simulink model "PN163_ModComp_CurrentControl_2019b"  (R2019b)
settings: Solver=VariableStepAuto  StartTime=0.0  StopTime=0.04  RelTol=1e-3
PostLoadFcn:
  | run('PN163_param.m');
model workspace (MAT data in the model file):
  CTRLPERIOD = [5e-05 2.5001e-05]
  global_cycle_delay = 1e-05
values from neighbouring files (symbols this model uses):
  C = 260e-6    (= 0.00026)    [PN163_param.m]
  fs = 20e3    (= 20000)    [PN163_param.m]
  ki = 1/Ti1    (= 165)    [PN163_param.m]
  kp = Tn1/Ti1    (= 18.75)    [PN163_param.m]
  Lb = 2.5e-3    (= 0.0025)    [PN163_param.m]
  Rb = 22e-3    (= 0.022)    [PN163_param.m]
  Rload = 5    [PN163_param.m]
  SAMPLEPERIOD = [Ts Ts*phase]    [PN163_param.m]
  Ts = 1/fs    (= 5e-05)    [PN163_param.m]
  Vb = 100    [PN163_param.m]
undefined symbols (not defined in the file or in its folder): A, AXI4, bit, code, DiscIntNeverNeededParam, HLS, N, Stream, Top, width, xc7z030fbg676
libraries: ModelComposer x42, powerlib x24, powerlib_meascontrol x2

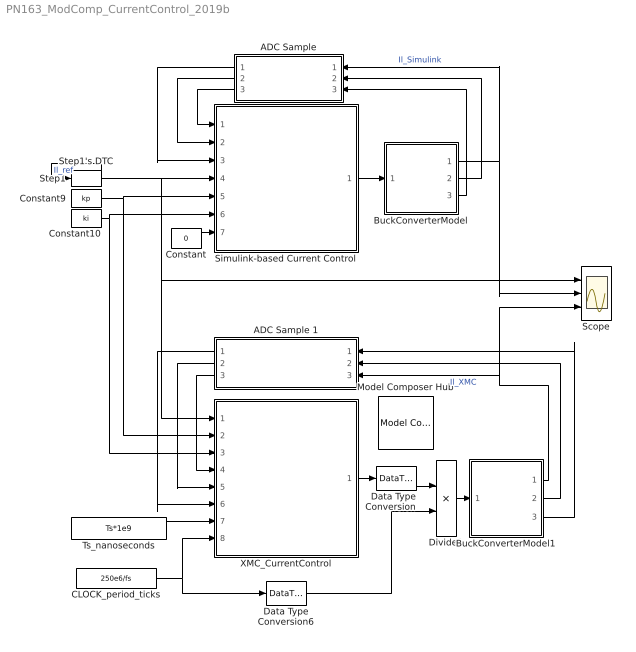
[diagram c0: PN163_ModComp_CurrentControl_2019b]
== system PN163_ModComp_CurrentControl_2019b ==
  ADC Sample : Subsystem
  ADC Sample 1 : Subsystem
  BuckConverterModel : Subsystem
  BuckConverterModel1 : Subsystem
  CLOCK_period_ticks : Constant  Value=250e6/fs  OutDataTypeStr=uint16  SampleTime=SAMPLEPERIOD
  Constant : Constant  Value=0  OutDataTypeStr=Inherit: Inherit via back propagation
  Constant10 : Constant  Value=ki  OutDataTypeStr=single  SampleTime=SAMPLEPERIOD
  Constant9 : Constant  Value=kp  OutDataTypeStr=single  SampleTime=SAMPLEPERIOD
  Data Type Conversion : DataTypeConversion  OutDataTypeStr=double
  Data Type Conversion6 : DataTypeConversion  OutDataTypeStr=double
  Divide1 : Product  Inputs=*/
  Model Composer Hub : ModelComposer/Model Composer Hub  CodeGeneration=off  SubsystemName=XMC_CurrentControl  TargetDirectory=C:/KB/PN163/Generated/Code  ExportType=HLS C++ code  IpVendor=xilinx.com  IpLibrary=hls  IpVersion=1.0  IpHWLanguage=Verilog  AieCompilerOptions={}  CreateTestbench=off  TestbenchStackSize=10  RunAieSim=off  AieSimTimeout=50000  LaunchVitisAnalyzer=off  RunX86Sim=off  X86SimTimeout=10  ProjDevice=xc7z030fbg676-3  ProjDevicePart=xc7z030fbg676-3  SamplePeriod=-1  ClockFrequency=250  DataPathParallelism=1
  Scope : Scope  NumInputPorts=3
  Simulink-based Current Control : Subsystem
  Step1 : Step  Time=0.02  Before=3  After=5  SampleTime=SAMPLEPERIOD
  Step1's DTC : DataTypeConversion
  Ts_nanoseconds : Constant  Value=Ts*1e9  OutDataTypeStr=uint32  SampleTime=SAMPLEPERIOD
  XMC_CurrentControl : Subsystem
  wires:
  BuckConverterModel/1(I) -> ADC Sample/1(Il_in), Scope/2  "Il_Simulink"
  Ts_nanoseconds/1 -> XMC_CurrentControl/7(Ts)
  Constant9/1 -> XMC_CurrentControl/2(Kp), Simulink-based Current Control/5(Kp)
  Constant10/1 -> Simulink-based Current Control/6(Ki), XMC_CurrentControl/3(Ki)
  XMC_CurrentControl/1(duty_cycle_ticks) -> Data Type Conversion/1
  Divide1/1 -> BuckConverterModel1/1(duty_cycle)
  ADC Sample 1/3(I_raw_int16) -> XMC_CurrentControl/4(Il_raw)
  ADC Sample 1/2(Vin_raw_int16) -> XMC_CurrentControl/5(Vin_raw)
  ADC Sample 1/1(Vout_raw_int16) -> XMC_CurrentControl/6(Vout_raw)
  BuckConverterModel1/3(Vout) -> ADC Sample 1/1(Vout_single)
  BuckConverterModel1/2(Vin) -> ADC Sample 1/2(Vin_single)
  BuckConverterModel1/1(I) -> Scope/3, ADC Sample 1/3(I_single)  "Il_XMC"
  Data Type Conversion/1 -> Divide1/1
  CLOCK_period_ticks/1 -> Data Type Conversion6/1, XMC_CurrentControl/8(CLOCK_period)
  Data Type Conversion6/1 -> Divide1/2
  Constant/1 -> Simulink-based Current Control/7(reset)
  Simulink-based Current Control/1(duty_cycle) -> BuckConverterModel/1(duty_cycle)
  BuckConverterModel/2(Vin) -> ADC Sample/2(Vin_in)
  BuckConverterModel/3(Vout) -> ADC Sample/3(vout_in)
  ADC Sample/3(Vout) -> Simulink-based Current Control/1(Vout)
  ADC Sample/2(Vin) -> Simulink-based Current Control/2(Vin)
  ADC Sample/1(Il) -> Simulink-based Current Control/3(Il)
  Step1/1 -> Step1's DTC/1  "Il_ref"
  Step1's DTC/1 -> XMC_CurrentControl/1(Il_ref), Scope/1, Simulink-based Current Control/4(I_ref)

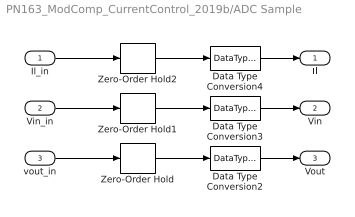
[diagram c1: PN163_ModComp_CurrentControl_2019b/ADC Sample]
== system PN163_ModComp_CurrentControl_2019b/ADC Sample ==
  Il_in : Inport
  Vin_in : Inport  Port=2
  vout_in : Inport  Port=3
  Data Type Conversion2 : DataTypeConversion  OutDataTypeStr=single
  Data Type Conversion3 : DataTypeConversion  OutDataTypeStr=single
  Data Type Conversion4 : DataTypeConversion  OutDataTypeStr=single
  Zero-Order Hold : ZeroOrderHold  SampleTime=SAMPLEPERIOD
  Zero-Order Hold1 : ZeroOrderHold  SampleTime=SAMPLEPERIOD
  Zero-Order Hold2 : ZeroOrderHold  SampleTime=SAMPLEPERIOD
  Il : Outport
  Vin : Outport  Port=2
  Vout : Outport  Port=3
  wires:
  Il_in/1 -> Zero-Order Hold2/1
  Data Type Conversion2/1 -> Vout/1
  Zero-Order Hold2/1 -> Data Type Conversion4/1
  Zero-Order Hold/1 -> Data Type Conversion2/1
  Vin_in/1 -> Zero-Order Hold1/1
  Zero-Order Hold1/1 -> Data Type Conversion3/1
  vout_in/1 -> Zero-Order Hold/1
  Data Type Conversion4/1 -> Il/1
  Data Type Conversion3/1 -> Vin/1

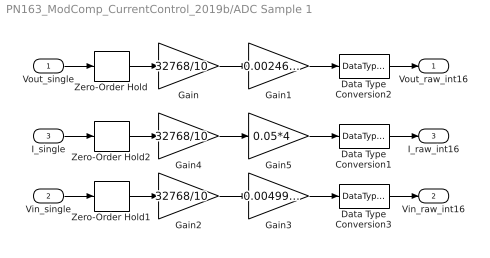
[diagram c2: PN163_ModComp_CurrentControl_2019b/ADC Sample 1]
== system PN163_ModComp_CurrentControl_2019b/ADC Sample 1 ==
  Vout_single : Inport
  Vin_single : Inport  Port=2
  I_single : Inport  Port=3
  Data Type Conversion1 : DataTypeConversion  OutDataTypeStr=int16
  Data Type Conversion2 : DataTypeConversion  OutDataTypeStr=int16
  Data Type Conversion3 : DataTypeConversion  OutDataTypeStr=int16
  Gain : Gain  Gain=32768/10
  Gain1 : Gain  Gain=0.00246*4
  Gain2 : Gain  Gain=32768/10
  Gain3 : Gain  Gain=0.00499*4
  Gain4 : Gain  Gain=32768/10
  Gain5 : Gain  Gain=0.05*4
  Zero-Order Hold : ZeroOrderHold  SampleTime=SAMPLEPERIOD
  Zero-Order Hold1 : ZeroOrderHold  SampleTime=SAMPLEPERIOD
  Zero-Order Hold2 : ZeroOrderHold  SampleTime=SAMPLEPERIOD
  Vout_raw_int16 : Outport
  Vin_raw_int16 : Outport  Port=2
  I_raw_int16 : Outport  Port=3
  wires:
  Vout_single/1 -> Zero-Order Hold/1
  Zero-Order Hold/1 -> Gain/1
  Gain/1 -> Gain1/1
  Data Type Conversion2/1 -> Vout_raw_int16/1
  Gain1/1 -> Data Type Conversion2/1
  Data Type Conversion3/1 -> Vin_raw_int16/1
  Gain3/1 -> Data Type Conversion3/1
  Zero-Order Hold1/1 -> Gain2/1
  Vin_single/1 -> Zero-Order Hold1/1
  Gain2/1 -> Gain3/1
  Gain4/1 -> Gain5/1
  I_single/1 -> Zero-Order Hold2/1
  Zero-Order Hold2/1 -> Gain4/1
  Gain5/1 -> Data Type Conversion1/1
  Data Type Conversion1/1 -> I_raw_int16/1

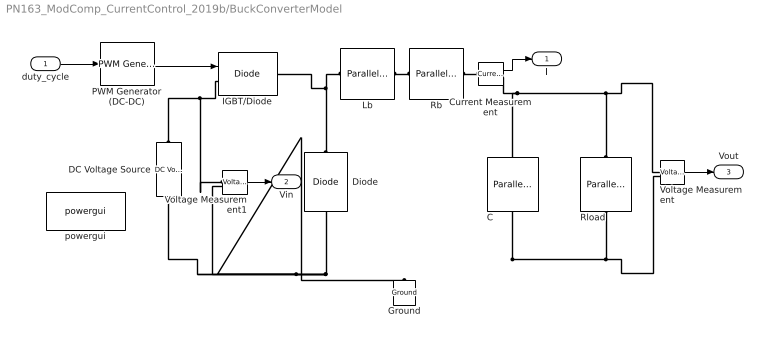
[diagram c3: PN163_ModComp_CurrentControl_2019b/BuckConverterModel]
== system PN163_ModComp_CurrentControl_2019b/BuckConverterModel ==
  duty_cycle : Inport
  C : powerlib/Elements/Parallel RLC Branch  LConnTagsString=a  RConnTagsString=__new0  BranchType=C  Resistance=5  Inductance=1e-3  SetiL0=off  InitialCurrent=0  Capacitance=C  Setx0=off  InitialVoltage=0  Measurements=None
  Current Measurement : powerlib/Measurements/Current Measurement  PhasorSimulation=off  OutputType=Complex  PSBequivalent=0
  DC Voltage Source : powerlib/Electrical Sources/DC Voltage Source  Amplitude=Vb  Measurements=Voltage
  Diode : powerlib/Power Electronics/Diode  Ron=0.001  Lon=0  Vf=0.8  IC=0  UseSnubber=0  Rs=500  Cs=250e-9  Measurements=off
  Ground : powerlib/Elements/Ground  LConnTagsString=a
  IGBT/Diode : powerlib/Power Electronics/IGBT//Diode  Ron=1e-3  Rs=1e5  Cs=inf  Measurements=off
  Lb : powerlib/Elements/Parallel RLC Branch  LConnTagsString=a  RConnTagsString=__new0  BranchType=L  Resistance=5  Inductance=Lb  SetiL0=off  InitialCurrent=0  Capacitance=1e-6  Setx0=off  InitialVoltage=0  Measurements=None
  PWM Generator (DC-DC) : powerlib_meascontrol/Pulse & Signal Generators/PWM Generator (DC-DC)  Fsw=fs  Ts=0
  Rb : powerlib/Elements/Parallel RLC Branch  LConnTagsString=a  RConnTagsString=__new0  BranchType=R  Resistance=Rb  Inductance=1e-3  SetiL0=off  InitialCurrent=0  Capacitance=1e-6  Setx0=off  InitialVoltage=0  Measurements=None
  Rload : powerlib/Elements/Parallel RLC Branch  LConnTagsString=a  RConnTagsString=__new0  BranchType=R  Resistance=Rload  Inductance=1e-3  SetiL0=off  InitialCurrent=0  Capacitance=1e-6  Setx0=off  InitialVoltage=0  Measurements=None
  Voltage Measurement : powerlib/Measurements/Voltage Measurement  PhasorSimulation=off  OutputType=Complex  PSBequivalent=0
  Voltage Measurement1 : powerlib/Measurements/Voltage Measurement  PhasorSimulation=off  OutputType=Complex  PSBequivalent=0
  powergui : powerlib/powergui  Priority=1  SimulationMode=Continuous  SampleTime=50e-6  frequency=60  Iterations=50  frequencyindice=0  Pbase=100e6  ErrMax=1e-4  UnitsV=kV  UnitsW=MW  buscounter=0  FunctionMessages=off  echomessages=off  EnableUseOfTLC=off  CurrentSourceSwitches=off  DisableSnubberDevices=off  DisableRonSwitches=off  DisableVfSwitches=off  DisplayEquations=off  AutomaticDiscreteSolvers=off  SolverType=Tustin/Backward Euler (TBE)  Interpol=off  ExternalGateDelay=off  methode=off  Ts=100  x0status=blocks  SPID=on  SwTol=0  HookPort=off  NonlinearTolerance=1e-4  nMaxIteration=100  ContinueOnMaxIteration=off  RestoreLinks=warning  ResistiveCurrentMeasurement=off  Frange=[0:2:500]  Ylog=off  Xlog=on  ShowGrid=off  save=off  variable=ZData  structure=0  ZoomFFT=off  StartTime=0.0  cycles=1  DisplayStyle=1  fundamental=60  FreqAxis=off  MaxFrequency=1000  frequencyindicesteady=1  RmsSteady=1  display=off
  I : Outport
  Vin : Outport  Port=2
  Vout : Outport  Port=3
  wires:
  duty_cycle/1 -> PWM Generator (DC-DC)/1
  Current Measurement/1 -> I/1
  Voltage Measurement1/1 -> Vin/1
  Voltage Measurement/1 -> Vout/1
  PWM Generator (DC-DC)/1 -> IGBT/Diode/1
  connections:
  Rload/RConn1 -- C/RConn1 -- DC Voltage Source/LConn1 -- Voltage Measurement1/LConn2 -- Diode/LConn1 -- Ground/LConn1 -- Voltage Measurement/LConn2
  DC Voltage Source/RConn1 -- IGBT/Diode/LConn1 -- Voltage Measurement1/LConn1
  Rload/LConn1 -- Current Measurement/RConn1 -- C/LConn1 -- Voltage Measurement/LConn1
  Lb/RConn1 -- Rb/LConn1
  Diode/RConn1 -- Lb/LConn1 -- IGBT/Diode/RConn1
  Rb/RConn1 -- Current Measurement/LConn1

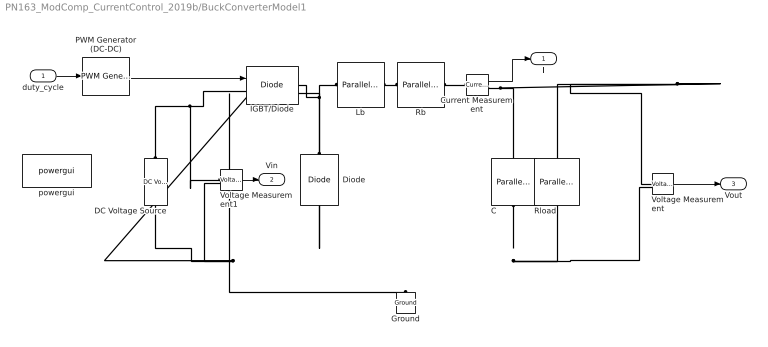
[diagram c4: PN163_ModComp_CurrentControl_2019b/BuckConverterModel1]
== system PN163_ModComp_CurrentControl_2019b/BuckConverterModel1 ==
  duty_cycle : Inport
  C : powerlib/Elements/Parallel RLC Branch  LConnTagsString=a  RConnTagsString=__new0  BranchType=C  Resistance=5  Inductance=1e-3  SetiL0=off  InitialCurrent=0  Capacitance=C  Setx0=off  InitialVoltage=0  Measurements=None
  Current Measurement : powerlib/Measurements/Current Measurement  PhasorSimulation=off  OutputType=Complex  PSBequivalent=0
  DC Voltage Source : powerlib/Electrical Sources/DC Voltage Source  Amplitude=Vb  Measurements=Voltage
  Diode : powerlib/Power Electronics/Diode  Ron=0.001  Lon=0  Vf=0.8  IC=0  UseSnubber=0  Rs=500  Cs=250e-9  Measurements=off
  Ground : powerlib/Elements/Ground  LConnTagsString=a
  IGBT/Diode : powerlib/Power Electronics/IGBT//Diode  Ron=1e-3  Rs=1e5  Cs=inf  Measurements=off
  Lb : powerlib/Elements/Parallel RLC Branch  LConnTagsString=a  RConnTagsString=__new0  BranchType=L  Resistance=5  Inductance=Lb  SetiL0=off  InitialCurrent=0  Capacitance=1e-6  Setx0=off  InitialVoltage=0  Measurements=None
  PWM Generator (DC-DC) : powerlib_meascontrol/Pulse & Signal Generators/PWM Generator (DC-DC)  Fsw=fs  Ts=0
  Rb : powerlib/Elements/Parallel RLC Branch  LConnTagsString=a  RConnTagsString=__new0  BranchType=R  Resistance=Rb  Inductance=1e-3  SetiL0=off  InitialCurrent=0  Capacitance=1e-6  Setx0=off  InitialVoltage=0  Measurements=None
  Rload : powerlib/Elements/Parallel RLC Branch  LConnTagsString=a  RConnTagsString=__new0  BranchType=R  Resistance=Rload  Inductance=1e-3  SetiL0=off  InitialCurrent=0  Capacitance=1e-6  Setx0=off  InitialVoltage=0  Measurements=None
  Voltage Measurement : powerlib/Measurements/Voltage Measurement  PhasorSimulation=off  OutputType=Complex  PSBequivalent=0
  Voltage Measurement1 : powerlib/Measurements/Voltage Measurement  PhasorSimulation=off  OutputType=Complex  PSBequivalent=0
  powergui : powerlib/powergui  Priority=1  SimulationMode=Continuous  SampleTime=50e-6  frequency=60  Iterations=50  frequencyindice=0  Pbase=100e6  ErrMax=1e-4  UnitsV=kV  UnitsW=MW  buscounter=0  FunctionMessages=off  echomessages=off  EnableUseOfTLC=off  CurrentSourceSwitches=off  DisableSnubberDevices=off  DisableRonSwitches=off  DisableVfSwitches=off  DisplayEquations=off  AutomaticDiscreteSolvers=off  SolverType=Tustin/Backward Euler (TBE)  Interpol=off  ExternalGateDelay=off  methode=off  Ts=100  x0status=blocks  SPID=on  SwTol=0  HookPort=off  NonlinearTolerance=1e-4  nMaxIteration=100  ContinueOnMaxIteration=off  RestoreLinks=warning  ResistiveCurrentMeasurement=off  Frange=[0:2:500]  Ylog=off  Xlog=on  ShowGrid=off  save=off  variable=ZData  structure=0  ZoomFFT=off  StartTime=0.0  cycles=1  DisplayStyle=1  fundamental=60  FreqAxis=off  MaxFrequency=1000  frequencyindicesteady=1  RmsSteady=1  display=off
  I : Outport
  Vin : Outport  Port=2
  Vout : Outport  Port=3
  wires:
  duty_cycle/1 -> PWM Generator (DC-DC)/1
  Current Measurement/1 -> I/1
  Voltage Measurement1/1 -> Vin/1
  Voltage Measurement/1 -> Vout/1
  PWM Generator (DC-DC)/1 -> IGBT/Diode/1
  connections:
  C/RConn1 -- Rload/RConn1 -- Voltage Measurement/LConn2 -- Voltage Measurement1/LConn2 -- DC Voltage Source/LConn1 -- Diode/LConn1 -- Ground/LConn1
  DC Voltage Source/RConn1 -- Voltage Measurement1/LConn1 -- IGBT/Diode/LConn1
  Current Measurement/RConn1 -- C/LConn1 -- Voltage Measurement/LConn1 -- Rload/LConn1
  Lb/RConn1 -- Rb/LConn1
  Diode/RConn1 -- IGBT/Diode/RConn1 -- Lb/LConn1
  Rb/RConn1 -- Current Measurement/LConn1

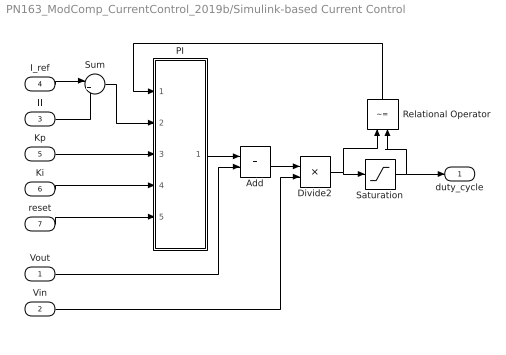
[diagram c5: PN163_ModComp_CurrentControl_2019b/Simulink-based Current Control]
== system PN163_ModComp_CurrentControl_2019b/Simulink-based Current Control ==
  Vout : Inport
  Vin : Inport  Port=2
  Il : Inport  Port=3
  I_ref : Inport  Port=4
  Kp : Inport  Port=5
  Ki : Inport  Port=6
  reset : Inport  Port=7
  Add : Sum
  Divide2 : Product  Inputs=*/
  PI : Subsystem
  Relational Operator : RelationalOperator  Operator=~=  OutDataTypeStr=boolean  RndMeth=Simplest
  Saturation : Saturate  UpperLimit=1  LowerLimit=0
  Sum : Sum  Inputs=|+-
  duty_cycle : Outport
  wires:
  Saturation/1 -> duty_cycle/1, Relational Operator/2
  Divide2/1 -> Saturation/1, Relational Operator/1
  Add/1 -> Divide2/1
  Kp/1 -> PI/3(Kp)
  Il/1 -> Sum/2
  Sum/1 -> PI/2(err)
  Relational Operator/1 -> PI/1(sat)
  PI/1(y) -> Add/1
  Vout/1 -> Add/2
  Ki/1 -> PI/4(Ki)
  I_ref/1 -> Sum/1
  Vin/1 -> Divide2/2
  reset/1 -> PI/5(reset)

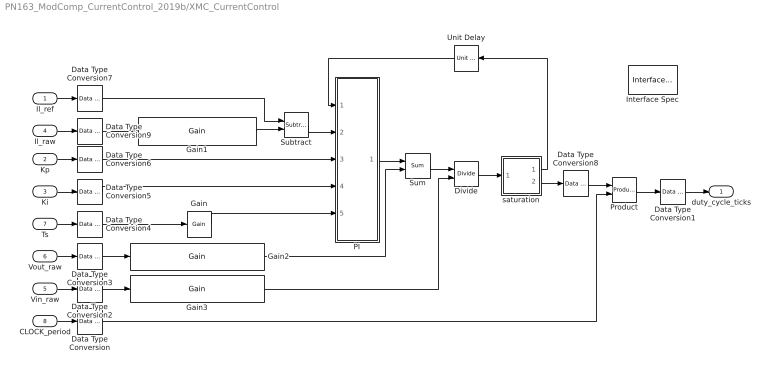
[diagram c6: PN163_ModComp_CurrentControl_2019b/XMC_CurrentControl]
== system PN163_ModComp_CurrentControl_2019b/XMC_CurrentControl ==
  Il_ref : Inport  OutDataTypeStr=single
  Kp : Inport  Port=2  OutDataTypeStr=single
  Ki : Inport  Port=3  OutDataTypeStr=single
  Il_raw : Inport  Port=4  OutDataTypeStr=int16
  Vin_raw : Inport  Port=5  OutDataTypeStr=int16
  Vout_raw : Inport  Port=6  OutDataTypeStr=int16
  Ts : Inport  Port=7  OutDataTypeStr=uint32
  CLOCK_period : Inport  Port=8  OutDataTypeStr=uint16
  Data Type Conversion : ModelComposer/Data Type Conversion  OutDataType=uint16  TypeExp=''  Signedness=Signed  WordLength=16  FractionalLength=0  RoundingMode=Truncation to minus infinity  OverflowMode=Wrap around
  Data Type Conversion1 : ModelComposer/Data Type Conversion  OutDataType=uint16  TypeExp=''  Signedness=Signed  WordLength=16  FractionalLength=0  RoundingMode=Truncation to minus infinity  OverflowMode=Wrap around  SaturateOnIntegerOverflow=on
  Data Type Conversion{2..7,9} (7 alike) : ModelComposer/Data Type Conversion  OutDataType=single  TypeExp=''  Signedness=Signed  WordLength=16  FractionalLength=0  RoundingMode=Truncation to minus infinity  OverflowMode=Wrap around
  Data Type Conversion8 : ModelComposer/Data Type Conversion  OutDataType=fixed  TypeExp=''  Signedness=Signed  WordLength=17  FractionalLength=16  RoundingMode=Truncation to minus infinity  OverflowMode=Saturation
  Divide : ModelComposer/Divide
  Gain : ModelComposer/Gain  Gain=1e-9  OutDataType=single  TypeExp=''  Signedness=Signed  WordLength=16  FractionalLength=0  RoundingMode=Truncation to minus infinity  OverflowMode=Wrap around  OutputTypeAsInput=on
  Gain1 : ModelComposer/Gain  Gain=(10/32768)/(0.05*4)  OutDataType=single  TypeExp=''  Signedness=Signed  WordLength=16  FractionalLength=0  RoundingMode=Truncation to minus infinity  OverflowMode=Wrap around  OutputTypeAsInput=on
  Gain2 : ModelComposer/Gain  Gain=(10/32768)/(0.00499*4)  OutDataType=single  TypeExp=''  Signedness=Signed  WordLength=16  FractionalLength=0  RoundingMode=Truncation to minus infinity  OverflowMode=Wrap around  OutputTypeAsInput=on
  Gain3 : ModelComposer/Gain  Gain=(10/32768)/(0.00499*4)  OutDataType=single  TypeExp=''  Signedness=Signed  WordLength=16  FractionalLength=0  RoundingMode=Truncation to minus infinity  OverflowMode=Wrap around  OutputTypeAsInput=on
  Interface Spec : ModelComposer/Interface Spec  Return=No block-level I/O protocol@@  InportInterfaces={'AXI4-Stream@@@N/A@N/A', 'AXI4-Stream@@@N/A@N/A', 'AXI4-Stream@@@N/A@N/A', 'AXI4-Stream@@@N/A@N/A', 'AXI4-Stream@@@N/A@N/A', 'AXI4-Stream@@@N/A@N/A', 'AXI4-Stream@@@N/A@N/A', 'No protocol@@@N/A@N/A'}  InportHandles={6.729000244140625000e+03, 6.730000244140625000e+03, 6.739000244140625000e+03, 6.740000244140625000e+03, 6.741000244140625000e+03, 6.742000244140625000e+03, 6.743000244140625000e+03, 6.744000244140625000e+03}  InportNames={'Il_ref', 'Kp', 'Ki', 'Il_raw', 'Vin_raw', 'Vout_raw', 'Ts', 'CLOCK_period'}  OutportInterfaces={'Valid Port@@@N/A@N/A'}  OutportHandles={7.009000244140625000e+03}  OutportNames={'duty_cycle_ticks'}  Mode=No block-level I/O protocol  InName1=Il_ref  InMode1=AXI4-Stream  InVFormat1=N/A  InVComponent1=N/A  InName2=Kp  InMode2=AXI4-Stream  InVFormat2=N/A  InVComponent2=N/A  InName3=Ki  InMode3=AXI4-Stream  InVFormat3=N/A  InVComponent3=N/A  InName4=Il_raw  InMode4=AXI4-Stream  InVFormat4=N/A  InVComponent4=N/A  InName5=Vin_raw  InMode5=AXI4-Stream  InVFormat5=N/A  InVComponent5=N/A  InName6=Vout_raw  InMode6=AXI4-Stream  InVFormat6=N/A  InVComponent6=N/A  InName7=Ts  InMode7=AXI4-Stream  InVFormat7=N/A  InVComponent7=N/A  InName8=CLOCK_period  InMode8=No protocol  InVFormat8=N/A  InVComponent8=N/A  OutName1=duty_cycle_ticks  OutMode1=Valid Port  OutVFormat1=N/A  OutVComponent1=N/A  OutName2=duty_cycle_B  OutMode2=No protocol  OutVFormat2=N/A  OutVComponent2=N/A  OutName3=duty_cycle_C  OutMode3=No protocol  OutVFormat3=N/A  OutVComponent3=N/A  OutMode4=Default  OutVFormat4=N/A  OutVComponent4=N/A  OutMode5=Default  OutVFormat5=N/A  OutVComponent5=N/A  OutMode6=Default  OutVFormat6=N/A  OutVComponent6=N/A  OutMode7=Default  OutVFormat7=N/A  OutVComponent7=N/A  OutMode8=Default  OutVFormat8=N/A  OutVComponent8=N/A
  PI : Subsystem
  Product : ModelComposer/Product
  Subtract : ModelComposer/Subtract
  Sum : ModelComposer/Sum
  Unit Delay : ModelComposer/Unit Delay  InitialCondition=0
  saturation : Subsystem
  duty_cycle_ticks : Outport
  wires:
  Data Type Conversion6/1 -> PI/3(Kp)
  Data Type Conversion5/1 -> PI/4(Ki)
  Gain/1 -> PI/5(Ts)
  Data Type Conversion4/1 -> Gain/1
  Ts/1 -> Data Type Conversion4/1
  Vout_raw/1 -> Data Type Conversion3/1
  Sum/1 -> Divide/1
  Vin_raw/1 -> Data Type Conversion2/1
  PI/1(y) -> Sum/1
  CLOCK_period/1 -> Data Type Conversion/1
  Ki/1 -> Data Type Conversion5/1
  Kp/1 -> Data Type Conversion6/1
  Il_ref/1 -> Data Type Conversion7/1
  saturation/1(sat) -> Unit Delay/1
  Data Type Conversion1/1 -> duty_cycle_ticks/1
  Product/1 -> Data Type Conversion1/1
  Data Type Conversion/1 -> Product/2
  Divide/1 -> saturation/1(in)
  saturation/2(out) -> Data Type Conversion8/1
  Data Type Conversion8/1 -> Product/1
  Il_raw/1 -> Data Type Conversion9/1
  Data Type Conversion7/1 -> Subtract/1
  Data Type Conversion9/1 -> Gain1/1
  Subtract/1 -> PI/2(err)
  Data Type Conversion3/1 -> Gain2/1
  Data Type Conversion2/1 -> Gain3/1
  Gain1/1 -> Subtract/2
  Gain2/1 -> Sum/2
  Gain3/1 -> Divide/2
  Unit Delay/1 -> PI/1(sat)

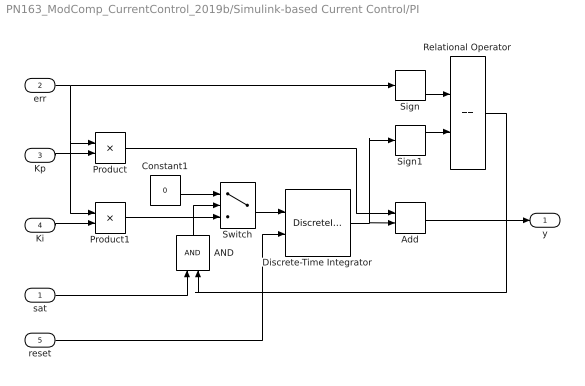
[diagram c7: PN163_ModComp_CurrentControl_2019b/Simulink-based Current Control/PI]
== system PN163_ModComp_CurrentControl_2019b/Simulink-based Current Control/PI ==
  sat : Inport
  err : Inport  Port=2
  Kp : Inport  Port=3
  Ki : Inport  Port=4
  reset : Inport  Port=5
  AND : Logic  AllPortsSameDT=off  OutDataTypeStr=boolean
  Add : Sum
  Constant1 : Constant  Value=0
  Discrete-Time Integrator : DiscreteIntegrator  ExternalReset=level  SampleTime=-1  ICPrevOutput=DiscIntNeverNeededParam  ICPrevScaledInput=DiscIntNeverNeededParam
  Product : Product
  Product1 : Product
  Relational Operator : RelationalOperator  Operator===  OutDataTypeStr=boolean  RndMeth=Simplest
  Sign : Signum
  Sign1 : Signum
  Switch : Switch  Criteria=u2 ~= 0
  y : Outport
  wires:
  Ki/1 -> Product1/2
  Relational Operator/1 -> AND/2
  sat/1 -> AND/1
  Add/1 -> y/1
  Product1/1 -> Switch/3
  Product/1 -> Add/1
  err/1 -> Sign/1, Product/1, Product1/1
  Kp/1 -> Product/2
  Discrete-Time Integrator/1 -> Add/2, Sign1/1
  AND/1 -> Switch/2
  Constant1/1 -> Switch/1
  Sign1/1 -> Relational Operator/2
  Sign/1 -> Relational Operator/1
  reset/1 -> Discrete-Time Integrator/2
  Switch/1 -> Discrete-Time Integrator/1

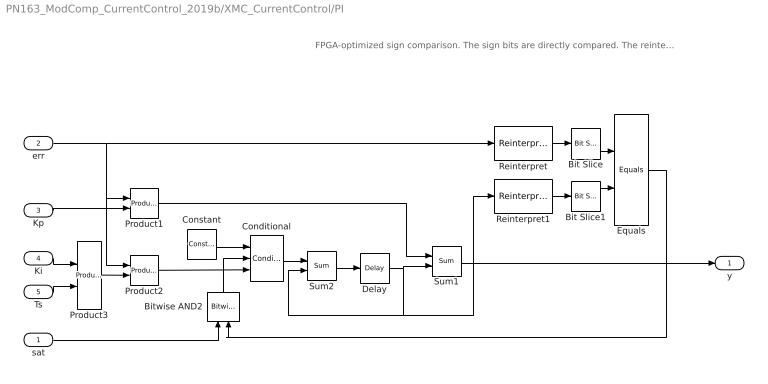
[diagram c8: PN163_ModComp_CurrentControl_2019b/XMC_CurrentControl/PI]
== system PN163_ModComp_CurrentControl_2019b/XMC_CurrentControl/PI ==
  note: FPGA-optimized sign comparison. The sign bits are directly compared. The reinterpret blocks are required because the bit slice does not support floating point inputs.
  sat : Inport
  err : Inport  Port=2
  Kp : Inport  Port=3
  Ki : Inport  Port=4
  Ts : Inport  Port=5
  Bit Slice : ModelComposer/Bit Slice  RangeSpec=Top bit + width  RangeWidth=1  TopRangeAnchor=Most Significant Bit  TopRangeOffset=0  BotRangeAnchor=Least Significant Bit  BotRangeOffset=0
  Bit Slice1 : ModelComposer/Bit Slice  RangeSpec=Top bit + width  RangeWidth=1  TopRangeAnchor=Most Significant Bit  TopRangeOffset=0  BotRangeAnchor=Least Significant Bit  BotRangeOffset=0
  Bitwise AND2 : ModelComposer/Bitwise AND
  Conditional : ModelComposer/Conditional  Condition=C ~= 0  Threshold=0.00
  Constant : ModelComposer/Constant  Value=0  SampleTime=inf  OutDataType=single  TypeExp=''  Signedness=Signed  WordLength=16  FractionalLength=0  RoundingMode=Truncation to minus infinity  OverflowMode=Wrap around
  Delay : ModelComposer/Delay  Latency=1
  Equals : ModelComposer/Equals
  Product1 : ModelComposer/Product
  Product2 : ModelComposer/Product
  Product3 : ModelComposer/Product
  Reinterpret : ModelComposer/Reinterpret  OutDataType=uint32  TypeExp=''  Signedness=Signed  wordLenHolder=inherited  FractionalLength=0
  Reinterpret1 : ModelComposer/Reinterpret  OutDataType=uint32  TypeExp=''  Signedness=Signed  wordLenHolder=inherited  FractionalLength=0
  Sum1 : ModelComposer/Sum
  Sum2 : ModelComposer/Sum
  y : Outport
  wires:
  Product3/1 -> Product2/2
  Ts/1 -> Product3/2
  Ki/1 -> Product3/1
  Equals/1 -> Bitwise AND2/2
  sat/1 -> Bitwise AND2/1
  Sum1/1 -> y/1
  Product2/1 -> Conditional/3
  Bit Slice/1 -> Equals/1
  Product1/1 -> Sum1/1
  Bit Slice1/1 -> Equals/2
  err/1 -> Reinterpret/1, Product1/1, Product2/1
  Kp/1 -> Product1/2
  Reinterpret/1 -> Bit Slice/1
  Reinterpret1/1 -> Bit Slice1/1
  Delay/1 -> Sum1/2, Reinterpret1/1, Sum2/2
  Sum2/1 -> Delay/1
  Bitwise AND2/1 -> Conditional/2
  Constant/1 -> Conditional/1
  Conditional/1 -> Sum2/1

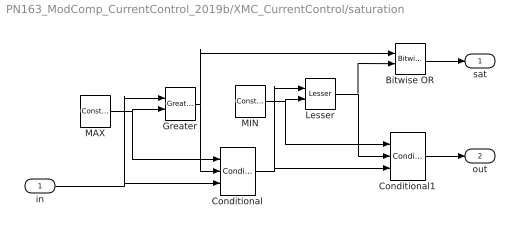
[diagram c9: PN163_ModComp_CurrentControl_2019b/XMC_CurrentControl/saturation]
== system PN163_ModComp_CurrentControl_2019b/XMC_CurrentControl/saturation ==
  in : Inport
  Bitwise OR : ModelComposer/Bitwise OR
  Conditional : ModelComposer/Conditional  Condition=C ~= 0  Threshold=0.00
  Conditional1 : ModelComposer/Conditional  Condition=C ~= 0  Threshold=0.00
  Greater : ModelComposer/Greater
  Lesser : ModelComposer/Lesser
  MAX : ModelComposer/Constant  Value=1  SampleTime=-1  OutDataType=single  TypeExp=''  Signedness=Signed  WordLength=16  FractionalLength=0  RoundingMode=Truncation to minus infinity  OverflowMode=Wrap around
  MIN : ModelComposer/Constant  Value=0  SampleTime=-1  OutDataType=single  TypeExp=''  Signedness=Signed  WordLength=16  FractionalLength=0  RoundingMode=Truncation to minus infinity  OverflowMode=Wrap around
  sat : Outport
  out : Outport  Port=2
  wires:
  Bitwise OR/1 -> sat/1
  Lesser/1 -> Conditional1/2, Bitwise OR/2
  MIN/1 -> Conditional1/1, Lesser/2
  MAX/1 -> Conditional/1, Greater/2
  Greater/1 -> Conditional/2, Bitwise OR/1
  in/1 -> Greater/1, Conditional/3
  Conditional1/1 -> out/1
  Conditional/1 -> Lesser/1, Conditional1/3
